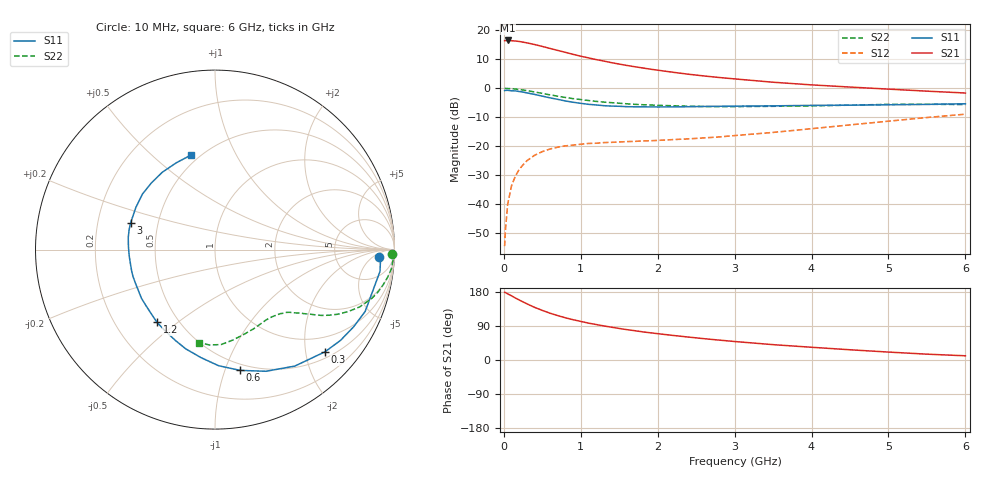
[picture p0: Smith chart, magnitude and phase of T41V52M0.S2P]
! Infineon Technologies  Discrete & RF Semiconductors
! BFR182T
! Si NPN RF Bipolar Junction Transistor in SC75
! VCE = 1.5 V  IC = 2 mA
! Common Emitter S-Parameters:  October  1999
# GHz  S  MA  R  50
!  f  S11  S21  S12  S22
! GHz  MAG  ANG  MAG  ANG  MAG  ANG  MAG  ANG
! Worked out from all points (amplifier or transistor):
!   36 points, 10 MHz to 6 GHz, reference 50 ohm
!   highest |S21| = 16.5 dB at 50 MHz (marker M1)
!   |S21| within 3 dB of that: start of sweep to 636.3 MHz
!   unconditionally stable (mu >= 1): 1.927 GHz to 4.435 GHz
!   at 250 MHz: K = 0.14, MSG = 21.1 dB, |S12| = -26.4 dB
!   at 1.4 GHz: K = 0.79, MSG = 13.7 dB, |S12| = -18.6 dB
!   at 6 GHz: K = 0.85, MSG = 3.7 dB, |S12| = -8.9 dB
!   lowest NFmin = 1.10 dB at 450 MHz
!   S11 on the Smith chart (normalised r, x): 10 MHz: 18, -9; 300 MHz: 0.63, -2.40; 600 MHz: 0.44, -1.13; 1.2 GHz: 0.38, -0.42; 3 GHz: 0.35, +0.14; 6 GHz: 0.45, +0.67
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0.01  0.9158 -2.5  6.678 178.4  0.0019 87.1  0.9892 -1.4
0.02  0.9237 -1.8  6.658 178.1  0.0035 82.0  0.9996 -1.3
0.05  0.9273 -7.5  6.708 174.5  0.0101 86.3  0.9939 -3.2
0.1  0.9091 -14.4  6.633 169.4  0.0209 82.9  0.9883 -6.3
0.15  0.9048 -22.4  6.564 163.6  0.0307 76.7  0.973 -9.3
0.2  0.8838 -29.2  6.442 158.3  0.0401 74.6  0.9562 -12.0
0.3  0.8365 -42.9  6.092 148.2  0.0566 67.1  0.9154 -17.2
0.4  0.7866 -55.6  5.707 138.9  0.0703 60.3  0.8671 -21.6
0.5  0.7353 -67.2  5.292 130.9  0.0812 55.3  0.8192 -24.9
0.6  0.6872 -78.3  4.887 123.5  0.09 51.3  0.7742 -27.7
0.8  0.6068 -97.4  4.185 111.4  0.1021 45.5  0.6979 -31.7
0.9  0.5766 -106.4  3.864 106.3  0.1051 43.5  0.6654 -33.1
1.1  0.5309 -121.7  3.359 97.3  0.1123 40.7  0.6176 -35.4
1.2  0.5184 -128.6  3.137 93.6  0.1132 39.6  0.5962 -36.5
1.4  0.4952 -141.0  2.774 86.5  0.1173 38.9  0.5672 -38.4
1.6  0.4836 -152.4  2.485 80.1  0.1209 39.0  0.542 -40.1
2.2  0.4795 -176.1  1.896 64.8  0.1309 42.7  0.5014 -46.5
3  0.4933 162.6  1.457 48.8  0.1535 49.8  0.4849 -56.5
3.5  0.4997 151.8  1.277 40.5  0.174 53.7  0.4907 -63.9
4.5  0.5133 133.8  1.054 27.0  0.2346 56.9  0.5136 -78.8
5.5  0.5296 114.0  0.896 15.4  0.3146 54.6  0.5322 -93.3
6  0.5431 104.4  0.832 11.1  0.3588 51.6  0.526 -99.9
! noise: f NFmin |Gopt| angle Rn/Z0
0.45  1.1  0.42  29  0.36
0.9  1.2  0.4  58  0.3
1.8  1.85  0.32  126  0.22
